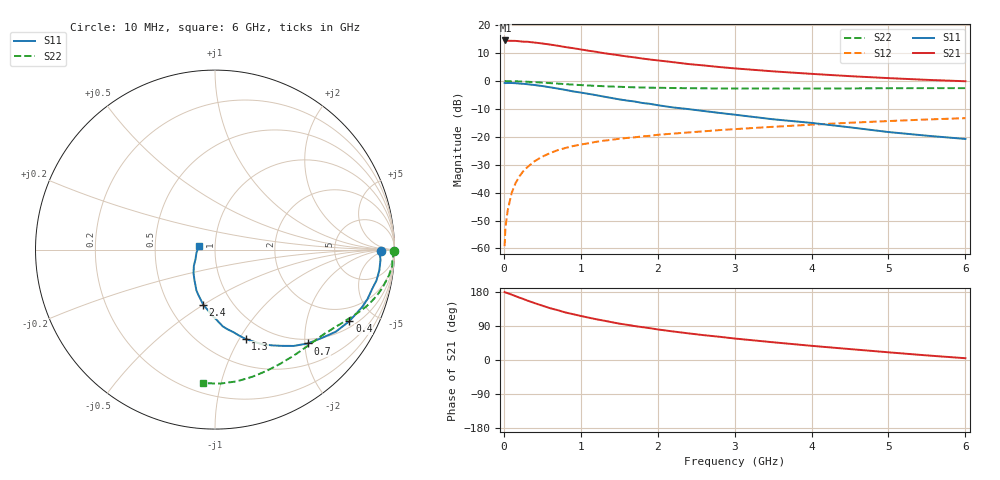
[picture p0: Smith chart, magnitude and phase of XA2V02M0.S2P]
! SIEMENS Discrete & RF Semiconductors
! BFY180
! Si NPN RF Bipolar Junction Transistor in MICRO-X
! VCE = 2 V  IC = 2 mA
! Common Emitter S-Parameters:  May  1997
# GHz  S  MA  R  50
!  f  S11  S21  S12  S22
! GHz  MAG  ANG  MAG  ANG  MAG  ANG  MAG  ANG
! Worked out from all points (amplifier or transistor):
!   36 points, 10 MHz to 6 GHz, reference 50 ohm
!   highest |S21| = 14.6 dB at 20 MHz (marker M1)
!   |S21| within 3 dB of that: start of sweep to 952.6 MHz
!   unconditionally stable (mu >= 1): 2.458 GHz to end of sweep
!   at 250 MHz: K = 0.14, MSG = 23.3 dB, |S12| = -32.4 dB
!   at 1.4 GHz: K = 0.74, MSG = 15.3 dB, |S12| = -21.1 dB
!   at 6 GHz: K = 1.09, MAG = 4.8 dB, |S12| = -13.3 dB
!   S11 on the Smith chart (normalised r, x): 10 MHz: 26, -3; 400 MHz: 1.26, -3.60; 700 MHz: 0.91, -2.06; 1.3 GHz: 0.77, -1.06; 2.4 GHz: 0.73, -0.50; 6 GHz: 0.84, +0.03
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0.01  0.926 -0.6  5.245 179.3  0.0011 81.4  0.9967 -0.3
0.02  0.9188 -1.3  5.34 178.3  0.0023 98.4  0.9996 -0.7
0.05  0.9238 -3.6  5.272 176.3  0.0048 86.5  0.994 -1.7
0.1  0.9228 -7.2  5.258 172.6  0.0097 88.0  0.9896 -3.4
0.15  0.916 -10.8  5.246 168.7  0.0146 83.6  0.9918 -5.2
0.3  0.8801 -21.3  5.068 157.3  0.0282 76.9  0.9717 -9.9
0.4  0.8485 -28.0  4.897 150.1  0.0367 72.9  0.9562 -13.0
0.6  0.7733 -39.5  4.508 136.8  0.0511 66.0  0.9196 -18.2
0.7  0.7345 -45.4  4.298 131.5  0.0577 62.7  0.9004 -20.6
0.8  0.6935 -50.7  4.067 125.5  0.0632 60.4  0.8811 -22.7
0.9  0.6531 -55.2  3.887 120.9  0.0684 57.6  0.8635 -24.6
1.1  0.5901 -63.4  3.501 111.9  0.0768 54.0  0.8323 -28.0
1.3  0.5263 -71.1  3.164 103.9  0.0854 50.9  0.8086 -31.2
1.5  0.4696 -77.7  2.894 96.0  0.0925 48.6  0.7887 -34.1
1.7  0.4299 -84.2  2.656 89.6  0.0982 46.8  0.7717 -36.8
2.2  0.3366 -97.3  2.18 75.3  0.1144 42.7  0.7505 -43.5
2.4  0.3144 -102.1  2.018 70.3  0.12 41.3  0.7445 -46.2
3  0.2498 -114.5  1.687 56.7  0.1375 37.3  0.7353 -53.8
3.5  0.2066 -123.5  1.493 46.8  0.1515 34.1  0.7328 -60.3
4.5  0.1482 -142.6  1.224 28.8  0.179 26.8  0.7384 -73.6
5.5  0.1049 -170.1  1.051 12.1  0.2048 19.1  0.7471 -87.8
6  0.0918 167.0  0.992 4.7  0.2166 14.8  0.7469 -95.0
